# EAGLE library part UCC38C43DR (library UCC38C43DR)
Texas Instruments UCC38C43DR, PWM Current Mode Controller, 0.2 A, 1000 kHz 8-Pin SOIC Source: Datasheet
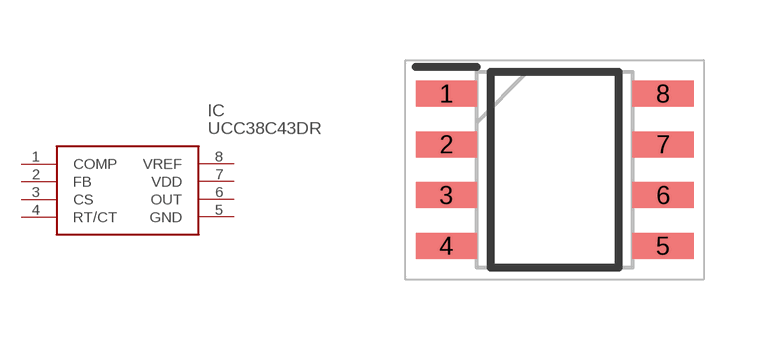
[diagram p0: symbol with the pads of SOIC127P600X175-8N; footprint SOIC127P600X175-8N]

Designator prefix IC

## UCC38C43DR (Description: Texas Instruments UCC38C43DR, PWM Current Mode Controller, 0.2 A, 1000 kHz 8-Pin SOIC; Height: 1.75mm; Manufacturer_Name: Texas Instruments; Manufacturer_Part_Number: UCC38C43DR; Mouser_Part_Number: 595-UCC38C43DR; Mouser_Price-Stock: https://www.mouser.co.uk/ProductDetail/Texas-Instruments/UCC38C43DR?qs=zqbRmZ%252BfZD8PGQXkq%2FjeEA%3D%3D)  [SOIC127P600X175-8N]
1  COMP
2  FB
3  CS
4  RT/CT
5  GND
6  OUT
7  VDD
8  VREF

## Footprint SOIC127P600X175-8N (pad centres in mm)
D(R-PDSO-G)
smd 1.528 x 0.65: 1 -2.711,1.905; 2 -2.711,0.635; 3 -2.711,-0.635; 4 -2.711,-1.905; 5 2.711,-1.905; 6 2.711,-0.635; 7 2.711,0.635; 8 2.711,1.905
